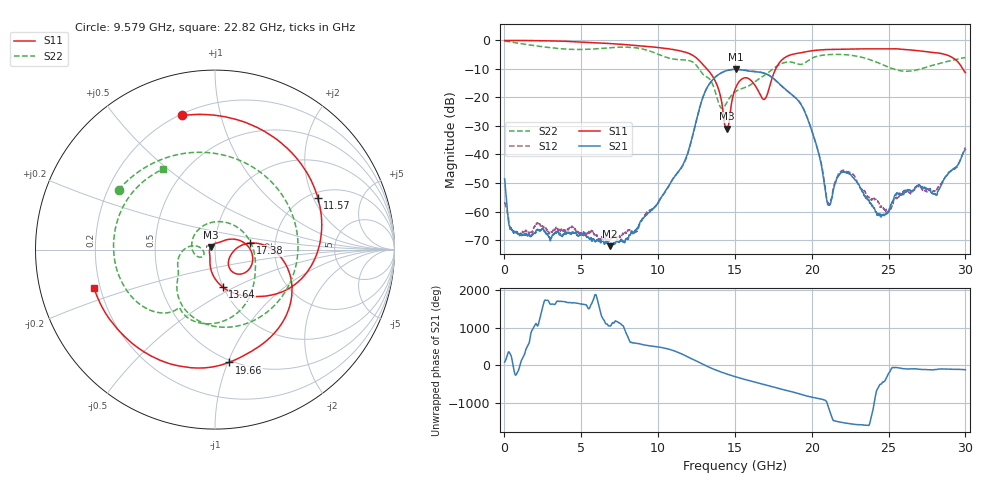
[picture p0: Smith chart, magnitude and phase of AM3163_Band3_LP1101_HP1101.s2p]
!Agilent Technologies,E8364B,MY43040894,A.07.50.67
!Agilent E8364B: A.07.50.67
!Date: Thursday, August 20, 2020 11:07:40
!Correction: S11(Full 2 Port(1,2))
!S21(Full 2 Port(1,2))
!S12(Full 2 Port(1,2))
!S22(Full 2 Port(1,2))
!S2P File: Measurements: S11, S21, S12, S22:
# Hz S  dB  R 50
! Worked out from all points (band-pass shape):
!   3201 points, 10 MHz to 30 GHz, reference 50 ohm
!   highest |S21| = -10.17 dB at 15.04 GHz (marker M1); lowest = -72.1 dB at 6.889 GHz (marker M2)
!   |S21| within 3 dB of the highest: 13.67 GHz to 17.47 GHz (3.802 GHz wide, 24.4 % of centre)
!   lowest |S11| = -31.0 dB at 14.46 GHz (marker M3), VSWR 1.06, Z = 47.6 + j1.43 ohm
!   |S11| at or under -10 dB: 13.18 GHz to 17.65 GHz (4.475 GHz wide, 29 % of centre); 29.82 GHz to end of sweep
!   |S22| runs from -23.9 to -0.2 dB; largest |S21 - S12| = 0.0069
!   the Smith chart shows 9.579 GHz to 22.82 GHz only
!   S11 on the Smith chart (normalised r, x): 9.579 GHz: 0.21, +0.76; 11.57 GHz: 2.21, +2.17; 13.64 GHz: 1.00, -0.44; 17.38 GHz: 1.49, +0.11; 19.66 GHz: 0.48, -1.01; 22.82 GHz: 0.18, -0.15
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1e7  -0.06 -2.0  -48.54 79.1  -56.68 -82.2  -0.23 -5.5
3.84875e8  -0.05 -10.3  -66.29 -69.3  -65.76 134.3  -0.55 -29.0
1.200228e9  -0.05 -32.1  -68.24 -157.3  -67.52 -24.8  -1.27 -83.4
2.587266e9  -0.14 -68.9  -66.93 -100.3  -65.97 165.9  -2.33 -164.0
5.014581e9  -0.58 -131.0  -67.86 -169.0  -67.77 -159.8  -3.21 68.9
6.888956e9  -1.14 -178.7  -72.15 -31.6  -69.85 109.5  -2.59 -35.5
8.097928e9  -1.59 148.6  -68.77 -31.8  -66.70 -91.0  -2.41 -108.1
9.578684e9  -2.28 103.7  -59.37 147.8  -59.37 144.5  -3.99 148.2
1.000979e10  -2.53 89.0  -56.99 124.3  -56.80 122.9  -4.88 112.3
1.156552e10  -3.85 26.8  -44.12 -67.3  -44.30 -68.6  -6.82 -34.0
1.363671e10  -13.42 -78.3  -13.34 -111.8  -13.26 -110.7  -16.65 173.6
1.446143e10  -30.98 147.9  -10.60 124.2  -10.63 124.5  -21.86 -150.8
1.5005e10  -17.24 23.4  -10.17 53.0  -10.22 54.0  -18.10 -177.1
1.504249e10  -16.73 20.6  -10.17 48.4  -10.21 49.4  -17.96 179.7
1.737608e10  -13.95 10.6  -12.77 146.1  -12.88 146.2  -10.43 -45.8
1.966282e10  -3.97 -82.9  -26.57 -101.9  -26.44 -100.9  -7.49 -124.8
2.000958e10  -3.64 -93.1  -31.80 -135.6  -31.70 -134.6  -6.29 -134.7
2.109672e10  -3.20 -122.1  -57.82 -53.0  -57.19 126.2  -5.01 -173.4
2.282114e10  -3.00 -162.4  -48.98 -141.9  -47.88 -146.9  -5.45 123.2
2.500479e10  -3.03 146.0  -59.88 143.2  -60.07 -97.2  -9.42 14.7
2.697288e10  -3.67 91.2  -50.73 -110.6  -51.49 -107.6  -10.18 -112.6
3e10  -11.36 -21.6  -38.31 -123.1  -37.51 -124.8  -6.02 121.1
